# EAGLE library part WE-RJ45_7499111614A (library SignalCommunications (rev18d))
Order Code 7499111614A Design THT xBase-T 10/100/1000 Base-T Ports 1x1 Application Standard HPLE Tab Position Up LED (Left-Right) GREEN/ORANGE-YELLOW EMI Fingers YES Details see: http://katalog.we-online.de/en/pbs/WE-LAN_RJ45/7499111614A? Updated by Yingchun Shan 2016-08-29 2016(C) Würth Elektronik
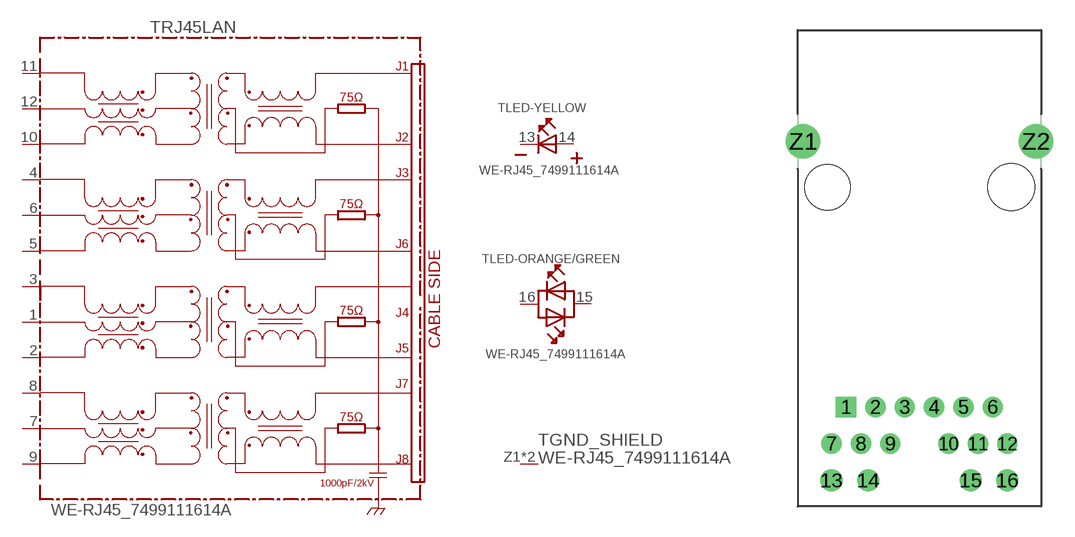
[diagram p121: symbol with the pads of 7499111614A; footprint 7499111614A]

Designator prefix T; gates RJ45LAN=7499111614A LED-YELLOW=LED-2PIN LED-ORANGE/GREEN=LED-DUAL GND_SHIELD=GND_PIN

## WE-RJ45_7499111614A (COMPANY-URL: http://www.we-online.de; CREATED-BY: Christin Zierenner; CREATED-DATE: AUG 2012; DATASHEET-URL: http://katalog.we-online.de/kataloge/eisos/media/pdf/7499111614A.pdf; MANUFACTURER: Würth Elektronik eiSos GmbH)  [7499111614A]
1  RJ45LAN:1
2  RJ45LAN:2
3  RJ45LAN:3
4  RJ45LAN:4
5  RJ45LAN:5
6  RJ45LAN:6
7  RJ45LAN:7
8  RJ45LAN:8
9  RJ45LAN:9
10  RJ45LAN:10
11  RJ45LAN:12
12  RJ45LAN:11
13  LED-YELLOW:K  pas
14  LED-YELLOW:A  pas
15  LED-ORANGE/GREEN:AK2  pas
16  LED-ORANGE/GREEN:AK1  pas
Z1  GND_SHIELD:1  pwr
Z2  GND_SHIELD:1  pwr

## Footprint 7499111614A (pad centres in mm)
MAX HEIGHT=13.87mm PORTS----1X1 LED --YES
drill 0.9 square: 1 -5.075,-15.24
drill 0.9: 2 -3.045,-15.24; 3 -1.015,-15.24; 4 1.015,-15.24; 5 3.045,-15.24; 6 5.075,-15.24; 7 -6.085,-17.78; 8 -4.055,-17.78; 9 -2.025,-17.78; 10 2.025,-17.78; 11 4.055,-17.78; 12 6.085,-17.78
drill 1.02: 13 -6.09,-20.32; 14 -3.55,-20.32; 15 3.55,-20.32; 16 6.09,-20.32
drill 1.6: Z1 -8.065,3.18; Z2 8.065,3.18
hole 3.25 at 6.35,0
hole 3.15 at -6.35,0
